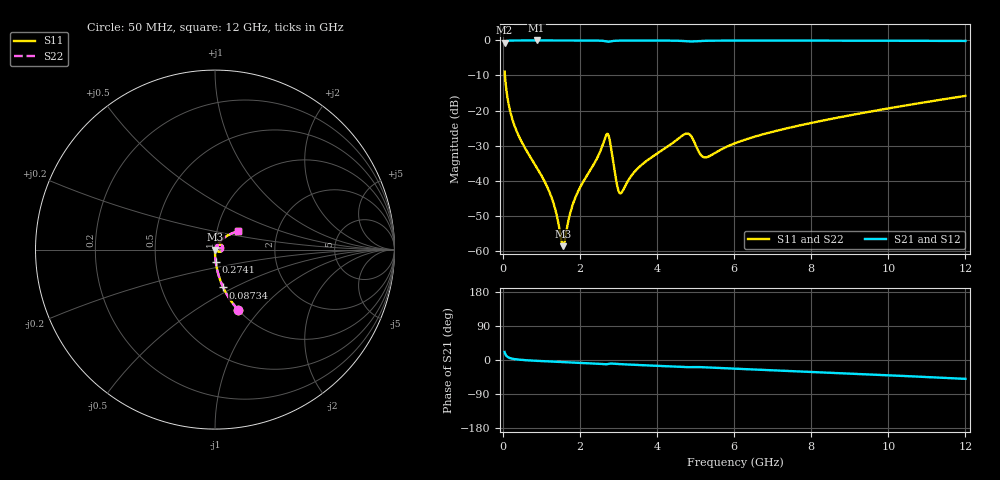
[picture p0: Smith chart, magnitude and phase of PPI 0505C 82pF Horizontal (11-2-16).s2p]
# MHz S MA R 50
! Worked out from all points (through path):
!   1601 points, 50 MHz to 12 GHz, reference 50 ohm
!   highest |S21| = -0.01 dB at 879 MHz (marker M1); lowest = -0.6 dB at 50 MHz (marker M2)
!   group delay of S21, straight-line fit = 11.8 ps
!   lowest |S11| = -58.7 dB at 1.566 GHz (marker M3), VSWR 1.00, Z = 50.1 - j0.0145 ohm
!   |S11| at or under -10 dB: 58 MHz to end of sweep
!   |S22| runs from -58.7 to -8.9 dB; largest |S21 - S12| = 0
!   S11 on the Smith chart (normalised r, x): 50 MHz: 1.00, -0.77; 87.34 MHz: 1.00, -0.44; 274.1 MHz: 1.00, -0.14; 12 GHz: 1.26, +0.26
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50  0.3606 -69.0  0.9324 21.0  0.9324 21.0  0.3606 -69.0
87.34375  0.2157 -77.8  0.9761 12.1  0.9761 12.1  0.2157 -77.8
169.5  0.1122 -83.9  0.9932 5.8  0.9932 5.8  0.1122 -83.9
274.0625  0.06847 -86.6  0.9971 3.0  0.9971 3.0  0.06847 -86.6
490.6562  0.03588 -88.6  0.9987 0.3  0.9987 0.3  0.03588 -88.6
879.0312  0.01559 -89.1  0.999 -2.2  0.999 -2.2  0.01559 -89.1
1274.875  0.005616 -83.7  0.9989 -4.2  0.9989 -4.2  0.005616 -83.7
1566.156  0.001165 -7.2  0.9987 -5.5  0.9987 -5.5  0.001165 -7.2
1805.156  0.004356 65.7  0.9986 -6.6  0.9986 -6.6  0.004356 65.7
2044.156  0.008739 71.7  0.9982 -7.7  0.9982 -7.7  0.008739 71.7
2701.406  0.04615 24.0  0.9617 -11.0  0.9617 -11.0  0.04615 24.0
2768.625  0.03951 -10.3  0.9603 -9.7  0.9603 -9.7  0.03951 -10.3
2955.344  0.009266 -20.8  0.9907 -10.3  0.9907 -10.3  0.009266 -20.8
3052.438  0.00659 16.0  0.9939 -10.9  0.9939 -10.9  0.00659 16.0
3478.156  0.01451 64.9  0.9966 -13.0  0.9966 -13.0  0.01451 64.9
4038.312  0.02501 66.4  0.9959 -15.6  0.9959 -15.6  0.02501 66.4
4762.781  0.04695 38.9  0.9739 -18.9  0.9739 -18.9  0.04695 38.9
5233.312  0.0215 32.9  0.9863 -19.2  0.9863 -19.2  0.0215 32.9
6025  0.03419 59.7  0.9946 -22.9  0.9946 -22.9  0.03419 59.7
8019.156  0.06687 55.7  0.994 -31.5  0.994 -31.5  0.06687 55.7
10013.31  0.1076 47.7  0.99 -40.4  0.99 -40.4  0.1076 47.7
12000  0.1618 38.8  0.982 -49.8  0.982 -49.8  0.1618 38.8
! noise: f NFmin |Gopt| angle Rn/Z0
50  0.0003752  0.8599  0.4296  0.0005734
1372  0.003875  0.6665  4.852  0.002226
2701  0.03228  0.9099  9.49  0.07826
4031  0.01192  0.6814  14.02  0.007141
5360  0.02258  0.7667  18.66  0.01918
6682  0.01559  0.6179  22.89  0.007318
8012  0.01648  0.5812  27.05  0.0068
9341  0.01816  0.5665  31.11  0.007055
1.067e+04  0.02012  0.561  35.04  0.007549
1.2e+04  0.02227  0.561  38.84  0.008189
